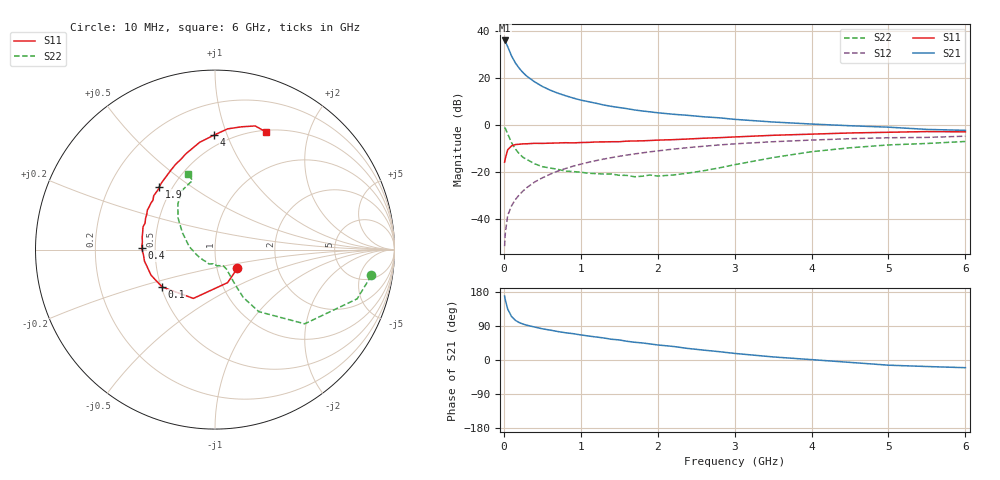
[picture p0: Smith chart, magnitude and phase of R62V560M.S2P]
! SIEMENS Small Signal Semiconductors
! BFR193
! Si NPN RF Bipolar Junction Transistor in SOT23
! VCE = 2.5 V  IC = 60 mA
! Common Emitter S-Parameters:  May  1996
# GHz  S  MA  R  50
!  f  S11  S21  S12  S22
! GHz  MAG  ANG  MAG  ANG  MAG  ANG  MAG  ANG
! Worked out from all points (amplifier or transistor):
!   36 points, 10 MHz to 6 GHz, reference 50 ohm
!   highest |S21| = 35.8 dB at 10 MHz (marker M1)
!   |S21| within 3 dB of that: start of sweep to 54.73 MHz
!   unconditionally stable (mu >= 1): 300.9 MHz to 2.076 GHz
!   at 250 MHz: K = 0.98, MSG = 25.1 dB, |S12| = -28.0 dB
!   at 1.4 GHz: K = 1.02, MAG = 9.9 dB, |S12| = -13.8 dB
!   at 6 GHz: K = 0.97, MSG = 1.2 dB, |S12| = -4.8 dB
!   S11 on the Smith chart (normalised r, x): 10 MHz: 1.25, -0.27; 100 MHz: 0.51, -0.24; 400 MHz: 0.42, +0.01; 1.9 GHz: 0.42, +0.38; 4 GHz: 0.42, +0.90; 6 GHz: 0.52, +1.39
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0.01  0.1627 -39.9  61.79 168.6  0.0027 79.5  0.8832 -9.4
0.02  0.197 -69.1  58.79 158.0  0.0053 77.5  0.8381 -19.1
0.05  0.2975 -113.9  45.65 134.5  0.0121 72.0  0.6486 -39.6
0.1  0.3607 -144.7  29.1 114.8  0.0193 69.5  0.423 -54.8
0.15  0.3839 -158.2  20.65 104.6  0.0262 72.4  0.3097 -59.4
0.2  0.3903 -166.1  15.87 98.8  0.033 73.3  0.2454 -59.9
0.25  0.3982 -170.7  12.83 94.8  0.04 74.2  0.2055 -60.1
0.3  0.3994 -175.4  10.75 91.7  0.0471 75.3  0.1852 -59.8
0.4  0.4084 178.8  8.203 87.0  0.0618 75.4  0.1505 -59.8
0.5  0.4068 174.1  6.561 82.4  0.0757 75.2  0.1309 -59.0
0.6  0.4115 170.3  5.488 79.0  0.0902 74.0  0.1225 -60.0
0.7  0.415 166.0  4.732 75.2  0.1051 73.2  0.115 -60.7
0.9  0.4167 159.3  3.729 69.5  0.1337 70.6  0.103 -62.7
1.1  0.4275 152.8  3.115 63.3  0.1618 67.9  0.0949 -69.7
1.4  0.4412 143.9  2.476 54.7  0.2031 63.5  0.0915 -82.3
1.9  0.4684 131.4  1.898 42.5  0.2694 55.8  0.087 -113.6
2.2  0.488 124.3  1.687 35.8  0.3076 51.0  0.0869 -135.9
3.5  0.6041 98.1  1.155 8.1  0.4413 30.0  0.2037 152.8
4  0.6389 90.3  1.046 1.0  0.4785 22.9  0.2712 139.4
4.5  0.6765 84.0  0.963 -6.3  0.5116 15.8  0.3285 129.0
5.5  0.7244 72.0  0.805 -17.2  0.5449 2.0  0.4053 108.0
6  0.7144 66.5  0.769 -20.3  0.5784 -2.1  0.4469 109.6
